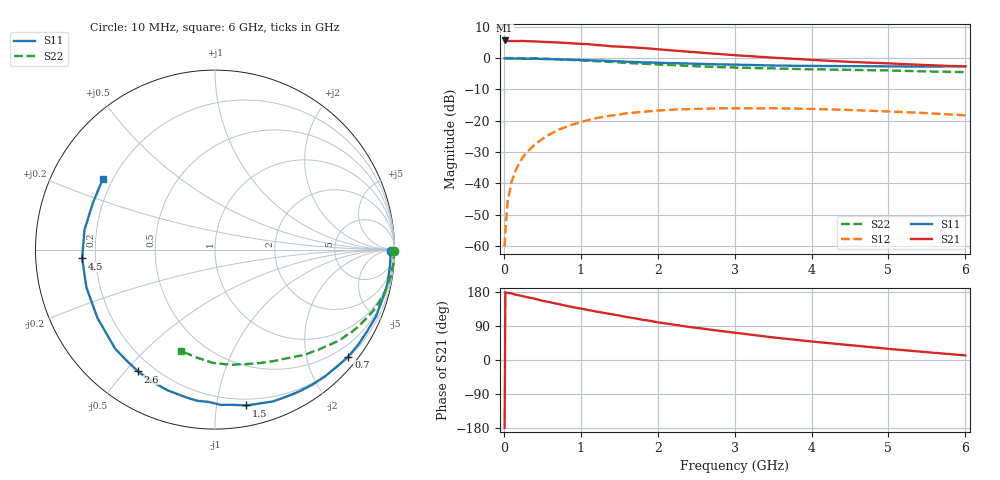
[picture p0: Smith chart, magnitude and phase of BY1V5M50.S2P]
! SIEMENS Small Signal Semiconductors
! BFY420
! Si NPN RF SIEGET Grounded Emitter Transistor in MICRO-X
! VCE = 1.5 V  IC = 0.5 mA
! Common Emitter S-Parameters:  October  1996
# GHz  S  MA  R  50
!  f  S11  S21  S12  S22
! GHz  MAG  ANG  MAG  ANG  MAG  ANG  MAG  ANG
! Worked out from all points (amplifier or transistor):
!   36 points, 10 MHz to 6 GHz, reference 50 ohm
!   highest |S21| = 5.6 dB at 10 MHz (marker M1)
!   |S21| within 3 dB of that: start of sweep to 2.096 GHz
!   unconditionally stable (mu >= 1): 4.729 GHz to end of sweep
!   at 250 MHz: K = 0.03, MSG = 18.5 dB, |S12| = -31.6 dB
!   at 1.4 GHz: K = 0.20, MSG = 11.0 dB, |S12| = -18.4 dB
!   at 6 GHz: K = 1.39, MAG = 4.1 dB, |S12| = -18.3 dB
!   S11 on the Smith chart (normalised r, x): 10 MHz: 77, -39; 700 MHz: 0.22, -2.83; 1.5 GHz: 0.15, -1.21; 2.6 GHz: 0.14, -0.54; 4.5 GHz: 0.15, -0.03; 6 GHz: 0.16, +0.28
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0.01  0.9794 -0.6  1.902 -179.2  0.001 102.7  0.9999 -0.3
0.02  0.9766 -1.4  1.897 178.8  0.0018 89.5  0.9966 -0.5
0.05  0.9785 -2.8  1.869 177.1  0.0051 89.1  0.9981 -1.4
0.1  0.9793 -5.7  1.868 175.9  0.0106 85.5  0.996 -2.9
0.15  0.9782 -8.4  1.86 172.3  0.0158 83.8  0.9963 -4.2
0.2  0.979 -11.2  1.863 170.7  0.0211 83.3  0.9946 -5.6
0.3  0.9718 -16.5  1.85 165.8  0.0316 79.5  0.991 -8.4
0.4  0.9715 -22.4  1.838 161.9  0.0413 76.2  0.9838 -11.2
0.5  0.9626 -27.9  1.81 156.3  0.0513 72.4  0.9753 -13.8
0.7  0.9526 -38.7  1.77 148.1  0.0706 65.2  0.954 -19.1
0.9  0.9351 -49.3  1.708 139.3  0.0875 58.1  0.9278 -24.1
1.1  0.9184 -59.7  1.659 131.8  0.1027 51.8  0.9032 -28.8
1.5  0.886 -78.6  1.518 117.4  0.1258 39.7  0.8492 -37.1
1.8  0.8493 -92.4  1.441 106.2  0.1383 32.0  0.8105 -42.6
2.2  0.8273 -108.5  1.314 93.6  0.15 22.4  0.7707 -49.6
2.6  0.803 -122.3  1.205 82.5  0.1552 14.8  0.7312 -55.6
3  0.7838 -135.2  1.108 72.1  0.1574 7.7  0.705 -61.5
3.5  0.7577 -149.9  1.011 59.6  0.158 0.3  0.6802 -68.2
4  0.7468 -163.6  0.934 48.9  0.1541 -5.9  0.66 -75.3
4.5  0.7418 -176.2  0.866 39.2  0.1484 -11.4  0.6467 -82.6
5.5  0.7284 159.0  0.77 20.6  0.1321 -18.8  0.6103 -99.4
6  0.7384 147.8  0.732 12.1  0.1218 -20.0  0.5953 -108.8
